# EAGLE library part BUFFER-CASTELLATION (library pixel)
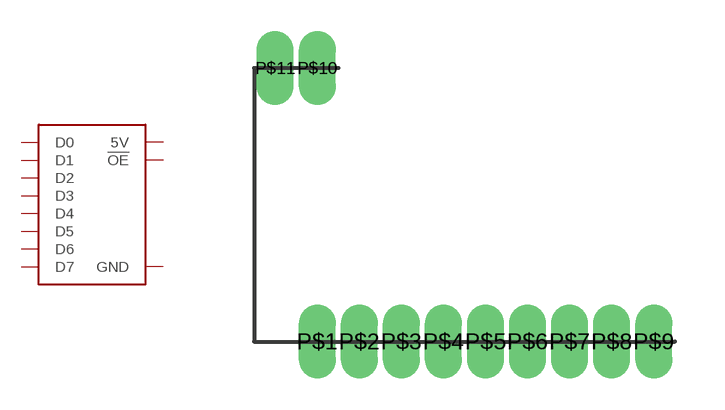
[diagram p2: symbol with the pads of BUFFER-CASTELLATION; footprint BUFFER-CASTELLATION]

Designator prefix -

## BUFFER-CASTELLATION  [BUFFER-CASTELLATION]
P$1  D0  in
P$2  D1  in
P$3  D2  in
P$4  D3  in
P$5  D4  in
P$6  D5  in
P$7  D6  in
P$8  D7  in
P$9  GND  in
P$10  !OE  in
P$11  5V  in

## Footprint BUFFER-CASTELLATION (pad centres in mm)
drill 0.61 pad 0.711 long: P$1 -4.445,-5.08; P$2 -3.175,-5.08; P$3 -1.905,-5.08; P$4 -0.635,-5.08; P$5 0.635,-5.08; P$6 1.905,-5.08; P$7 3.175,-5.08; P$8 4.445,-5.08; P$9 5.715,-5.08; P$10 -4.445,3.175; P$11 -5.715,3.175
